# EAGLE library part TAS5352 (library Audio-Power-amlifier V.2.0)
The TAS5352 is a high-performance, integrated stereo digital amplifier power stage designed to drive a 4-Ω bridge-tied load (BTL) at up to 125 W per channel with low harmonic distortion, low integrated noise, and low idle current.
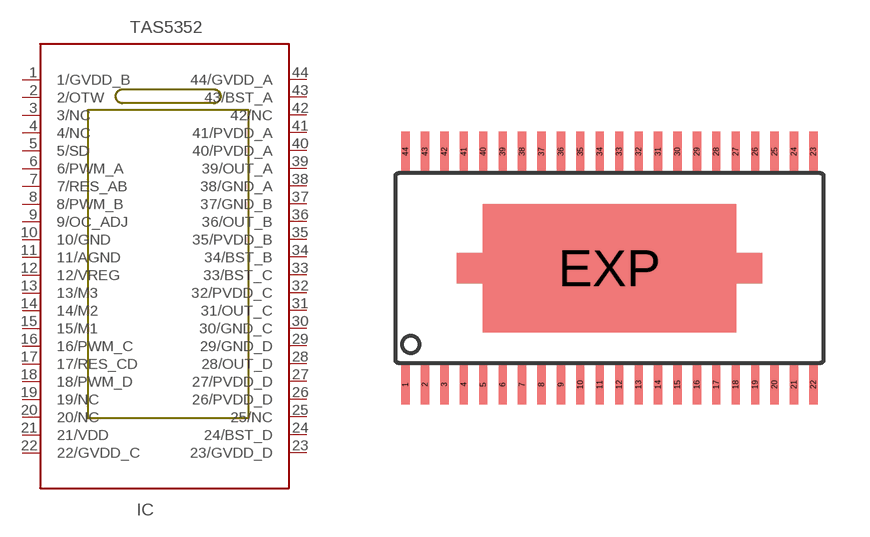
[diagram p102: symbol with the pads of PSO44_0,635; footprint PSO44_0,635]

Designator prefix IC

## TAS5352  [PSO44_0,635]
1  1/GVDD_B  pwr
2  2/OTW
3  3/NC  nc
4  4/NC  nc
5  5/SD
6  6/PWM_A  in
7  7/RES_AB  in
8  8/PWM_B  in
9  9/OC_ADJ  in
10  10/GND  pwr
11  11/AGND  pwr
12  12/VREG
13  13/M3
14  14/M2
15  15/M1
16  16/PWM_C  in
17  17/RES_CD  in
18  18/PWM_D  in
19  19/NC  nc
20  20/NC  nc
21  21/VDD  pwr
22  22/GVDD_C  pwr
23  23/GVDD_D  pwr
24  24/BST_D
25  25/NC  nc
26  26/PVDD_D  pwr
27  27/PVDD_D  pwr
28  28/OUT_D  out
29  29/GND_D  pwr
30  30/GND_C  pwr
31  31/OUT_C  out
32  32/PVDD_C  pwr
33  33/BST_C
34  34/BST_B
35  35/PVDD_B  pwr
36  36/OUT_B  out
37  37/GND_B  pwr
38  38/GND_A  pwr
39  39/OUT_A  out
40  40/PVDD_A  pwr
41  41/PVDD_A  pwr
42  42/NC  nc
43  43/BST_A
44  44/GVDD_A  pwr

## Footprint PSO44_0,635 (pad centres in mm)
smd 0.27 x 1.3: 1 -6.668,-3.81; 2 -6.032,-3.81; 3 -5.397,-3.81; 4 -4.763,-3.81; 5 -4.128,-3.81; 6 -3.493,-3.81; 7 -2.857,-3.81; 8 -2.223,-3.81; 9 -1.587,-3.81; 10 -0.953,-3.81; 11 -0.318,-3.81; 12 0.318,-3.81; 13 0.953,-3.81; 14 1.587,-3.81; 15 2.223,-3.81; 16 2.857,-3.81; 17 3.493,-3.81; 18 4.128,-3.81; 19 4.763,-3.81; 20 5.397,-3.81; 21 6.032,-3.81; 22 6.668,-3.81; 23 6.668,3.81; 24 6.032,3.81; 25 5.397,3.81; 26 4.763,3.81; 27 4.128,3.81; 28 3.493,3.81; 29 2.857,3.81; 30 2.223,3.81; 31 1.587,3.81; 32 0.953,3.81; 33 0.318,3.81; 34 -0.318,3.81; 35 -0.953,3.81; 36 -1.587,3.81; 37 -2.223,3.81; 38 -2.857,3.81; 39 -3.493,3.81; 40 -4.128,3.81; 41 -4.763,3.81; 42 -5.397,3.81; 43 -6.032,3.81; 44 -6.668,3.81
smd 8.3 x 4.2: EXP 0,0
